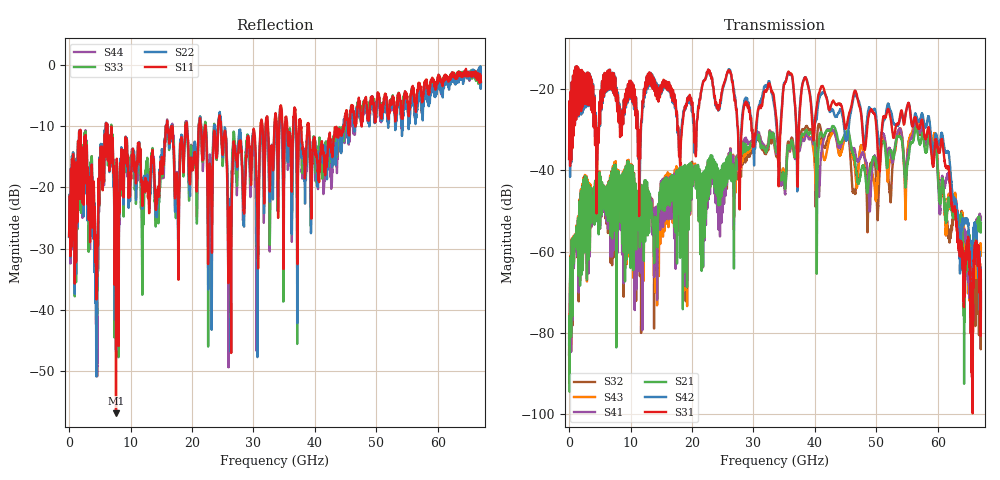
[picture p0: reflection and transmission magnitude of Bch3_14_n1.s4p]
!Agilent Technologies,N5247A,US51170199,A.09.90.13
!Agilent N5247A: A.09.90.13
!Date: Wednesday, October 17, 2018 17:56:40
!Correction: S11(Full 4 Port(1,2,3,4))
!S12(Full 4 Port(1,2,3,4))
!S13(Full 4 Port(1,2,3,4))
!S14(Full 4 Port(1,2,3,4))
!S21(Full 4 Port(1,2,3,4))
!S22(Full 4 Port(1,2,3,4))
!S23(Full 4 Port(1,2,3,4))
!S24(Full 4 Port(1,2,3,4))
!S31(Full 4 Port(1,2,3,4))
!S32(Full 4 Port(1,2,3,4))
!S33(Full 4 Port(1,2,3,4))
!S34(Full 4 Port(1,2,3,4))
!S41(Full 4 Port(1,2,3,4))
!S42(Full 4 Port(1,2,3,4))
!S43(Full 4 Port(1,2,3,4))
!S44(Full 4 Port(1,2,3,4))
!S4P File: Measurements: <S11,S12,S13,S14>,
!<S21,S22,S23,S24>,
!<S31,S32,S33,S34>,
!<S41,S42,S43,S44>:
# Hz S  dB  R 50
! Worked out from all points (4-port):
!   6701 points, 10 MHz to 67 GHz, reference 50 ohm
!   strongest paths, dB at 10 MHz, 16.76 GHz, 33.51 GHz, 50.25 GHz, 67 GHz:
!     S31: -37.2, -21.5, -24.2, -35.5, -70.0
!     S42: -37.2, -21.6, -25.3, -31.6, -67.0
!     S21: -82.9, -41.3, -33.9, -39.4, -53.0
!     S41: -85.3, -41.5, -34.0, -38.2, -51.7
!     S43: -81.2, -41.6, -34.2, -41.0, -59.2
!     S32: -85.4, -41.3, -35.0, -50.8, -74.2
!   lowest |S11| = -56.9 dB at 7.639 GHz (marker M1), VSWR 1.00, Z = 50.1 - j0.0522 ohm
!   |S11| at or under -10 dB: start of sweep to 5.979 GHz; 6.224 GHz to 15.74 GHz (9.519 GHz wide, 86.7 % of centre); 24.71 GHz to 31.15 GHz (6.447 GHz wide, 23.1 % of centre)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
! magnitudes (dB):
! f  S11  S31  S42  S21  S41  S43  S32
! 10 MHz  -28.0  -37.2  -37.2  -82.9  -85.3  -81.2  -85.4
! 2.46 GHz  -13.1  -16.2  -16.2  -56.8  -57.1  -57.3  -56.1
! 7.639 GHz  -56.9  -22.9  -22.3  -42.6  -43.1  -41.7  -43.3
! 55.18 GHz  -6.8  -23.5  -23.6  -37.4  -35.1  -33.6  -34.0
! 59.55 GHz  -3.2  -33.2  -31.9  -33.3  -33.2  -31.3  -32.4
! 64.44 GHz  -1.5  -62.2  -52.5  -63.6  -55.2  -57.8  -58.5
! 67 GHz  -2.7  -70.0  -67.0  -53.0  -51.7  -59.2  -74.2
